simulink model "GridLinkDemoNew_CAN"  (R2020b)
settings: Solver=FixedStepDiscrete  StartTime=0.0  StopTime=inf  RelTol=1e-3  EnableMultiTasking=on
InitFcn:
  | clc
  | close all
  | f_mod = 50000;
  | f_mod1 = 50*1e3; %[12 24 36 48 72 84 96 144]*1e3; %[18 36 48 72 84 96 144]*1e3;%
  | 
  | 
  | %%
  | 
  | 
  |             Tmod1 = 1/f_mod1;
  |             Tmod = 1/f_mod;
  |             Tc = Tmod1;
  |             Tsw=Tc;
  | 
  | warning off
  | f_sig = 60;
  | 
  | U_ac = 10;
  | U_dc = 20;
  | Ts= 0.01*Tsw;
  | 
  | Fc=50000
  | Fc1=1000
  | 
  | 
  | CounterCut_Outer=2000
  | 
  | 
  | INNER_PWM=1000
  | OUTER_PWM=50000
undefined symbols (not defined in the file): A, ADCIN0, ADCIN1, ADCINA0, ADCINB0, bit, Compare, conversion, DCAEVT1, DCAEVT1FILT, Digital, Down, ended, Event, Filtered, GPTRIP1SEL, GPTRIP2SEL, hex2dec, identifier, input, Module, Newinv, of, Single, SPS_EMT_TAPAS_2018b, Standard, start, Trip, TZ1, TZ2, Up, version, Zone
libraries: tiiqmathlib x63, c2802xlib x25, c2837xDlib x5, c280xlib x5, c28xdmclib x2, svdutilitieslib x1, c2000lib x1, canmsglib x1, simulink x1
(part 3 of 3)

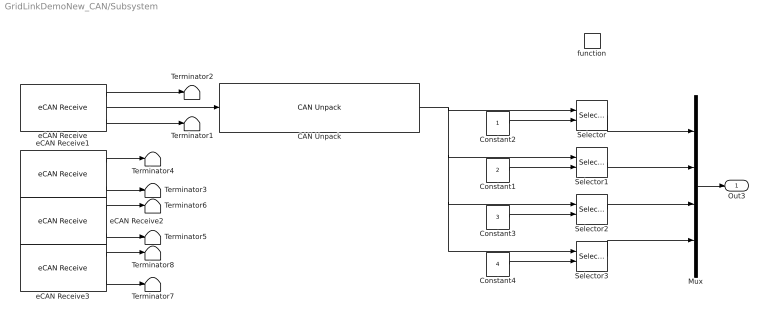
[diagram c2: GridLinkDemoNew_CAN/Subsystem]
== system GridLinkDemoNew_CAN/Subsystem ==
  function : TriggerPort  TriggerType=function-call  VariantControl=Variant
  CAN Unpack : canmsglib/CAN Unpack  MsgList=(none)  MsgName=CAN Msg  MsgIDType=Standard (11-bit identifier)  MsgIdentifier=hex2dec('01A')  MsgLength=4  SignalInfo={}  IDPort=off  TimestampPort=off  ErrorPort=off  RemotePort=off  LengthPort=off  StatusPort=off  ApplyMinMax=off
  Constant1 : Constant  Value=2  OutDataTypeStr=Inherit: Inherit via back propagation
  Constant2 : Constant  OutDataTypeStr=Inherit: Inherit via back propagation
  Constant3 : Constant  Value=3  OutDataTypeStr=Inherit: Inherit via back propagation
  Constant4 : Constant  Value=4  OutDataTypeStr=Inherit: Inherit via back propagation
  Mux : Mux
  Selector{,1..3} (4 alike) : Selector  InputPortWidth=4  IndexOptions=Index vector (port)  Indices=1  OutputSizes=1
  Terminator{1..8} (8 alike) : Terminator
  eCAN Receive : c280xlib/eCAN Receive  chipFamily=C280x  useModule=eCAN_B  mailboxNo=2  messageID=hex2dec('01A')  messageType=Standard (11-bit identifier)  sampleTime=-1  dataType=CAN_MESSAGE_TYPE  initValue=0  outputMessageLength=on  outputMessageTimeStamp=off  postInterrupt=on  interruptLine=0
  eCAN Receive1 : c280xlib/eCAN Receive  Commented=on  chipFamily=C280x  useModule=eCAN_B  mailboxNo=3  messageID=hex2dec('02A')  messageType=Standard (11-bit identifier)  sampleTime=-1  dataType=uint16  initValue=0  outputMessageLength=on  outputMessageTimeStamp=off  postInterrupt=on  interruptLine=0
  eCAN Receive2 : c280xlib/eCAN Receive  Commented=on  chipFamily=C280x  useModule=eCAN_B  mailboxNo=4  messageID=hex2dec('03A')  messageType=Standard (11-bit identifier)  sampleTime=-1  dataType=uint16  initValue=0  outputMessageLength=on  outputMessageTimeStamp=off  postInterrupt=on  interruptLine=0
  eCAN Receive3 : c280xlib/eCAN Receive  Commented=on  chipFamily=C280x  useModule=eCAN_B  mailboxNo=5  messageID=hex2dec('04A')  messageType=Standard (11-bit identifier)  sampleTime=-1  dataType=uint16  initValue=0  outputMessageLength=on  outputMessageTimeStamp=off  postInterrupt=on  interruptLine=0
  Out3 : Outport  VectorParamsAs1DForOutWhenUnconnected=off
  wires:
  eCAN Receive/1 -> Terminator2/1
  Constant2/1 -> Selector/2
  eCAN Receive/3 -> Terminator1/1
  eCAN Receive1/3 -> Terminator3/1
  Constant1/1 -> Selector1/2
  Selector1/1 -> Mux/2
  eCAN Receive1/1 -> Terminator4/1
  Constant3/1 -> Selector2/2
  eCAN Receive2/3 -> Terminator5/1
  Selector2/1 -> Mux/3
  eCAN Receive2/1 -> Terminator6/1
  Constant4/1 -> Selector3/2
  eCAN Receive3/3 -> Terminator7/1
  Selector3/1 -> Mux/4
  eCAN Receive3/1 -> Terminator8/1
  Mux/1 -> Out3/1
  Selector/1 -> Mux/1
  CAN Unpack/1 -> Selector3/1, Selector2/1, Selector1/1, Selector/1
  eCAN Receive/2 -> CAN Unpack/1

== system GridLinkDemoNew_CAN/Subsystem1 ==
  ePWM : c2802xlib/ePWM  PwmType=C2000_Type4  useModule=ePWM8  ePWMxLINKTBPRD=Not Linked  periodUnits=Clock cycles  timerSource=Specify via dialog  timerPeriod_clk=250  timerPeriod_sec=0.0001  tbshadow=Counter equals to zero  countingMode=Up-Down  phaseActiveEnable=Disable  phaseDirection=Count down after sync  phaseActive=0  synchronizationEnable=off  dcaevt1Sync=off  dcbevt1Sync=off  synchronizationOption=Disable  perSynchronizationOption=Counter equals to period (CTR=PRD)  clockPrescale=1  HSclockPrescale=1  enswap=off  ePWMxAStatus=on  ePWMxAactionLogic1=Do nothing  ePWMxAactionLogic2=Do nothing  ePWMxAactionLogic3=Set  ePWMxAactionLogic4=Clear  ePWMxAactionLogic5=Do nothing  ePWMxAactionLogic6=Do nothing  ePWMxACSFenable=off  ePWMxACSFvalue=Forcing disable  ePWMxASFreload=Zero  ePWMxBStatus=on  ePWMxBactionLogic1=Do nothing  ePWMxBactionLogic2=Do nothing  ePWMxBactionLogic3=Do nothing  ePWMxBactionLogic4=Do nothing  ePWMxBactionLogic5=Do nothing  ePWMxBactionLogic6=Do nothing  ePWMxBCSFenable=off  ePWMxBCSFvalue=Forcing disable  ePWMxBSFreload=Zero  ePWNxBOutWay=off  ePWMxLINKCMPA=Not Linked  CMPAUnits=Clock cycles  CMPASource=Specify via dialog  CMPAValue_per=50  CMPAValue_clk=10  enCMPAshadow=Counter equals to zero (CTR=Zero)  ePWMxLINKCMPB=Not Linked  CMPBUnits=Clock cycles  CMPBSource=Specify via dialog  CMPBValue_per=50  CMPBValue_clk=0  enCMPBshadow=Counter equals to zero (CTR=Zero)  ePWMxLINKCMPC=Not Linked  CMPCUnits=Clock cycles  CMPCSource=Specify via dialog  CMPCValue_per=50  CMPCValue_clk=0  enCMPCshadow=Counter equals to zero (CTR=Zero)  ePWMxLINKCMPD=Not Linked  CMPDUnits=Clock cycles  CMPDSource=Specify via dialog  CMPDValue_per=50  CMPDValue_clk=0  enCMPDshadow=Counter equals to zero (CTR=Zero)  enableDBePWMxA=off  enableDBePWMxB=off  enhalfcycle=off  DBpolarity=Active high (AH)  DBedgeDelay=Positive  DBSource_ePWMxA=ePWMxA  DBSource_ePWMxB=ePWMxA  DBPeriodUnits=Clock cycles  DBperiodSource=Specify via dialog  REDperiod=0  FEDperiod=0  REDperiod_sec=0  FEDperiod_sec=0  LoadModeDBRED=Immediate without using shadow  LoadModeDBFED=Immediate without using shadow  adcstartModuleA=off  adcrequestEventA=First event  adcstartEventA=Digital Compare Module A Event 1 start of conversion (DCAEVT1.soc)  adcstartEventA_type2=Counter equals to period (CTR=PRD)  adcstartModuleB=off  adcrequestEventB=First event  adcstartEventB=Counter equals to zero (CTR=Zero)  adcstartEventB_type2=Counter equals to zero (CTR=Zero)  intEn=on  intPrd=Third event  intSel=Counter equals to zero (CTR=Zero)  intSel_type2=Counter equals to zero (CTR=Zero)  hrpe=off  enHRPWM=off  HRPWM_LoadMode=Counter equals to period (CTR=PRD)  HRPWM_CTLMode=Duty or Period control mode  HRPWM_EDGMode=Both edge  hrpeb=off  enHRPWMB=off  HRPWM_LoadModeB=Counter equals to zero (CTR=ZERO)  HRPWM_CTLModeB=Duty or Period control mode  HRPWM_EDGModeB=Both edge  enHRDBRED=off  enHRDBFED=off  enSFO=on  enautoconv=on  chopperEnable=off  chopperFrequency=1  chopperFirstwidth=1  chopperDuty=12.5%  tripZonesource=Specify via dialog  tzselOSHT1=off  tzselOSHT2=off  tzselOSHT3=off  tzselOSHDCAEV1=off  tzselOSHDCBEV1=off  tzselCBC1=off  tzselCBC2=off  tzselCBC3=off  tzselCBCDCAEV2=off  tzselCBCDCBEV2=off  tzselOSHT4=off  tzselOSHT5=off  tzselOSHT6=off  tzselCBC4=off  tzselCBC5=off  tzselCBC6=off  enTzOstIntr=off  enTzCbcIntr=off  enTzDCAEVT1Intr=off  enTzDCAEVT2Intr=off  enTzDCBEVT1Intr=off  enTzDCBEVT2Intr=off  ePWMxAforced=No action  ePWMxBforced=No action  DCAEVT1forced=No action  DCBEVT1forced=No action  DCAEVT2forced=No action  DCBEVT2forced=No action  dcah=Trip Zone 1 input (TZ1)  dcal=Trip Zone 2 input (TZ2)  dcbh=Trip Zone 1 input (TZ1)  dcbl=Trip Zone 2 input (TZ2)  dcah_type2=GPTRIP1SEL/(TZ1)  dcal_type2=GPTRIP2SEL/(TZ2)  dcbh_type2=GPTRIP1SEL/(TZ1)  dcbl_type2=GPTRIP2SEL/(TZ2)  gendcaevt1=Event disabled  gendcaevt2=Event disabled  gendcbevt1=Event disabled  gendcbevt2=Event disabled  dcaevt1src=DCAEVT1 with sync  dcaevt2src=DCAEVT2 with sync  dcbevt1src=DCBEVT1 with sync  dcbevt2src=DCBEVT2 with sync  pulsesel=Counter equals to zero (CTR=Zero)  blankinv=off  blankoffset=0  blankwidth=0  evsrcsel=Filtered version of DCAEVT1 (DCAEVT1FILT)  encape=off

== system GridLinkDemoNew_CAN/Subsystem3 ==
  note: counter +=
  note: Reset counter
  function : TriggerPort  TriggerType=function-call  VariantControl=Variant
  Data Store Read1 : DataStoreRead  DataStoreName=CounterCut
  Data Store Read2 : DataStoreRead  DataStoreName=Counter
  If : If  NumInputs=2  IfExpression=u1 >= u2
  If Action Subsystem : Subsystem  TreatAsAtomicUnit=on
  If Action Subsystem1 : Subsystem  TreatAsAtomicUnit=on
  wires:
  Data Store Read2/1 -> If/1
  Data Store Read1/1 -> If/2
  If/2 -> If Action Subsystem1/Action
  If/1 -> If Action Subsystem/Action

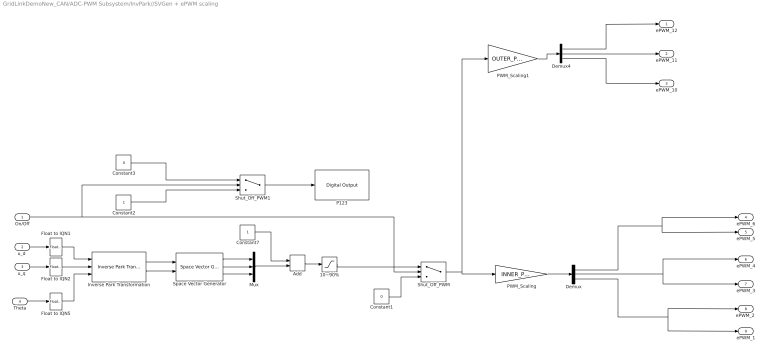
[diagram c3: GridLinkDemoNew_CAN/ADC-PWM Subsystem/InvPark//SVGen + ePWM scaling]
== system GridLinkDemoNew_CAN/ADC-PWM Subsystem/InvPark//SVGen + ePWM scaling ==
  On/Off : Inport
  "u_d " : Inport  Port=2
  "u_q " : Inport  Port=3
  Theta : Inport  Port=4
  10~90% : Saturate  UpperLimit=1.8  LowerLimit=0.2  OutDataTypeStr=Inherit: Inherit via back propagation
  Add : Sum
  Constant1 : Constant  Value=0  OutDataTypeStr=Inherit: Inherit via back propagation
  Constant2 : Constant  OutDataTypeStr=boolean
  Constant3 : Constant  Value=0  OutDataTypeStr=boolean
  Constant7 : Constant  OutDataTypeStr=Inherit: Inherit via back propagation
  Demux : Demux  Outputs=3
  Demux4 : Demux  Outputs=3
  Float to IQN1 : tiiqmathlib/Float to IQN  Q_value=16
  Float to IQN2 : tiiqmathlib/Float to IQN  Q_value=16
  Float to IQN5 : tiiqmathlib/Float to IQN  Q_value=16
  Inverse Park Transformation : c28xdmclib/Inverse Park Transformation
  Mux : Mux  Inputs=3
  P123 : c2837xDlib/Digital Output  GPIO_Number=GPIO112~GPIO119  GPIO_Bit0=off  GPIO_BIT0_Toggle=on  GPIO_Bit1=off  GPIO_BIT1_Toggle=on  GPIO_Bit2=off  GPIO_BIT2_Toggle=off  GPIO_Bit3=off  GPIO_BIT3_Toggle=off  GPIO_Bit4=off  GPIO_BIT4_Toggle=off  GPIO_Bit5=off  GPIO_BIT5_Toggle=on  GPIO_Bit6=off  GPIO_BIT6_Toggle=off  GPIO_Bit7=on  GPIO_BIT7_Toggle=off
  PWM_Scaling : Gain  Gain=INNER_PWM/2  ParamDataTypeStr=Inherit: Inherit from 'Gain'  OutDataTypeStr=Inherit: Inherit via back propagation
  PWM_Scaling1 : Gain  Gain=OUTER_PWM/2  ParamDataTypeStr=Inherit: Inherit from 'Gain'  OutDataTypeStr=Inherit: Inherit via back propagation
  Shut_Off_PWM : Switch  Criteria=u2 > Threshold  OutDataTypeStr=Inherit: Inherit via back propagation
  Shut_Off_PWM1 : Switch  Criteria=u2 > Threshold  OutDataTypeStr=Inherit: Inherit via back propagation
  Space Vector Generator : c28xdmclib/Space Vector Generator
  ePWM_12 : Outport  VectorParamsAs1DForOutWhenUnconnected=off
  ePWM_11 : Outport  Port=2  VectorParamsAs1DForOutWhenUnconnected=off
  ePWM_10 : Outport  Port=3  VectorParamsAs1DForOutWhenUnconnected=off
  ePWM_6 : Outport  Port=4  VectorParamsAs1DForOutWhenUnconnected=off
  ePWM_5 : Outport  Port=5  VectorParamsAs1DForOutWhenUnconnected=off
  ePWM_4 : Outport  Port=6  VectorParamsAs1DForOutWhenUnconnected=off
  ePWM_3 : Outport  Port=7  VectorParamsAs1DForOutWhenUnconnected=off
  "ePWM_2 " : Outport  Port=8  VectorParamsAs1DForOutWhenUnconnected=off
  ePWM_1 : Outport  Port=9  VectorParamsAs1DForOutWhenUnconnected=off
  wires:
  Float to IQN5/1 -> Inverse Park Transformation/3
  Theta/1 -> Float to IQN5/1
  "u_d "/1 -> Float to IQN1/1
  Space Vector Generator/3 -> Mux/3
  Space Vector Generator/2 -> Mux/2
  Space Vector Generator/1 -> Mux/1
  10~90%/1 -> Shut_Off_PWM/1
  Inverse Park Transformation/1 -> Space Vector Generator/1
  Mux/1 -> Add/2
  Add/1 -> 10~90%/1
  Inverse Park Transformation/2 -> Space Vector Generator/2
  Constant7/1 -> Add/1
  "u_q "/1 -> Float to IQN2/1
  Constant1/1 -> Shut_Off_PWM/3
  On/Off/1 -> Shut_Off_PWM1/2, Shut_Off_PWM/2
  Shut_Off_PWM1/1 -> P123/1
  Constant2/1 -> Shut_Off_PWM1/3
  Constant3/1 -> Shut_Off_PWM1/1
  Float to IQN1/1 -> Inverse Park Transformation/1
  Float to IQN2/1 -> Inverse Park Transformation/2
  Demux4/1 -> ePWM_12/1
  Demux4/3 -> ePWM_10/1
  Demux4/2 -> ePWM_11/1
  Shut_Off_PWM/1 -> PWM_Scaling/1, PWM_Scaling1/1
  PWM_Scaling1/1 -> Demux4/1
  PWM_Scaling/1 -> Demux/1
  Demux/1 -> ePWM_5/1, ePWM_6/1
  Demux/2 -> ePWM_4/1, ePWM_3/1
  Demux/3 -> "ePWM_2 "/1, ePWM_1/1

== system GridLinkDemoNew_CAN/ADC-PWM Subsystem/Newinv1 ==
  note: Input: uint16 Output: sfix32_En16
  note: voltage amplified by 100: e.g., 12 V => 1200
  A4 : Inport  OutDataTypeStr=uint16  PortDimensions=1
  A5 : Inport  Port=2  OutDataTypeStr=uint16  PortDimensions=1
  A6 : Inport  Port=3  OutDataTypeStr=uint16  PortDimensions=1
  B0 : Inport  Port=4  OutDataTypeStr=uint16  PortDimensions=1
  B1 : Inport  Port=5  OutDataTypeStr=uint16  PortDimensions=1
  B2 : Inport  Port=6  OutDataTypeStr=uint16  PortDimensions=1
  theta : Inport  Port=7
  Current scaling + Clarke/Park : Subsystem
  Voltage scaling + Clarke/Park : Subsystem
  Vd : Outport  PortDimensions=1  VectorParamsAs1DForOutWhenUnconnected=off
  Vq : Outport  Port=2  PortDimensions=1  VectorParamsAs1DForOutWhenUnconnected=off
  Id : Outport  Port=3  PortDimensions=1  VectorParamsAs1DForOutWhenUnconnected=off
  Iq : Outport  Port=4  PortDimensions=1  VectorParamsAs1DForOutWhenUnconnected=off
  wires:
  A5/1 -> Voltage scaling + Clarke/Park/2(V_ADC_2)
  Voltage scaling + Clarke/Park/2(V_q (ADC)) -> Vq/1
  B0/1 -> Current scaling + Clarke/Park/1(I_ADC_1)
  A4/1 -> Voltage scaling + Clarke/Park/1(V_ADC_1)
  A6/1 -> Voltage scaling + Clarke/Park/3(V_ADC_3)
  B2/1 -> Current scaling + Clarke/Park/3(I_ADC_3)
  B1/1 -> Current scaling + Clarke/Park/2(I_ADC_2)
  [theta] -> Voltage scaling + Clarke/Park/4(Theta)
  [theta] -> Current scaling + Clarke/Park/4(Theta)
  theta/1 -> [theta]
  Current scaling + Clarke/Park/1(I_d (ADC)) -> Id/1
  Current scaling + Clarke/Park/2(I_q (ADC)) -> Iq/1
  Voltage scaling + Clarke/Park/1(V_d (ADC)) -> Vd/1

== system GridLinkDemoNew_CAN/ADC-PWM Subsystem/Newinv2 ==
  note: Input: uint16 Output: sfix32_En16
  note: voltage amplified by 100: e.g., 12 V => 1200
  A4 : Inport  OutDataTypeStr=uint16  PortDimensions=1
  A5 : Inport  Port=2  OutDataTypeStr=uint16  PortDimensions=1
  A6 : Inport  Port=3  OutDataTypeStr=uint16  PortDimensions=1
  B0 : Inport  Port=4  OutDataTypeStr=uint16  PortDimensions=1
  B1 : Inport  Port=5  OutDataTypeStr=uint16  PortDimensions=1
  B2 : Inport  Port=6  OutDataTypeStr=uint16  PortDimensions=1
  theta : Inport  Port=7
  Current scaling + Clarke/Park : Subsystem
  Voltage scaling + Clarke/Park : Subsystem
  Vd : Outport  PortDimensions=1  VectorParamsAs1DForOutWhenUnconnected=off
  Vq : Outport  Port=2  PortDimensions=1  VectorParamsAs1DForOutWhenUnconnected=off
  Id : Outport  Port=3  PortDimensions=1  VectorParamsAs1DForOutWhenUnconnected=off
  Iq : Outport  Port=4  PortDimensions=1  VectorParamsAs1DForOutWhenUnconnected=off
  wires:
  A5/1 -> Voltage scaling + Clarke/Park/2(V_ADC_2)
  Voltage scaling + Clarke/Park/2(V_q (ADC)) -> Vq/1
  B0/1 -> Current scaling + Clarke/Park/1(I_ADC_1)
  A4/1 -> Voltage scaling + Clarke/Park/1(V_ADC_1)
  A6/1 -> Voltage scaling + Clarke/Park/3(V_ADC_3)
  B2/1 -> Current scaling + Clarke/Park/3(I_ADC_3)
  B1/1 -> Current scaling + Clarke/Park/2(I_ADC_2)
  [theta] -> Voltage scaling + Clarke/Park/4(Theta)
  [theta] -> Current scaling + Clarke/Park/4(Theta)
  theta/1 -> [theta]
  Current scaling + Clarke/Park/1(I_d (ADC)) -> Id/1
  Current scaling + Clarke/Park/2(I_q (ADC)) -> Iq/1
  Voltage scaling + Clarke/Park/1(V_d (ADC)) -> Vd/1

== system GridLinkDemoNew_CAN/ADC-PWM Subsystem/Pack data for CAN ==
  In1 : Inport
  In2 : Inport  Port=2
  In3 : Inport  Port=3
  In4 : Inport  Port=4
  Byte Pack2 : svdutilitieslib/Byte Pack  maskPackedDataType=uint16  datatypes={'uint16' 'uint16' 'uint16' 'uint16'}  byteAlign=2  blockPlatform=tic2000
  Data Type Conversion7 : DataTypeConversion  OutDataTypeStr=uint16
  Demux4 : Demux
  Mux6 : Mux
  Output : Outport  OutDataTypeStr=uint16  VectorParamsAs1DForOutWhenUnconnected=off
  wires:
  Mux6/1 -> Data Type Conversion7/1
  In1/1 -> Mux6/1
  Data Type Conversion7/1 -> Demux4/1
  In2/1 -> Mux6/2
  In4/1 -> Mux6/4
  In3/1 -> Mux6/3
  Byte Pack2/1 -> Output/1
  Demux4/1 -> Byte Pack2/1
  Demux4/2 -> Byte Pack2/2
  Demux4/3 -> Byte Pack2/3
  Demux4/4 -> Byte Pack2/4

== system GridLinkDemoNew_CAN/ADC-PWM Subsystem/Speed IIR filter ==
  Speed : Inport
  Add : Sum  Inputs=+-
  Add1 : Sum
  Constant1 : Constant  OutDataTypeStr=fixdt(1,32,16)
  Constant2 : Constant  Value=.01  OutDataTypeStr=fixdt(1,32,16)
  Product : Product
  Product1 : Product
  Unit Delay : UnitDelay  SampleTime=-1  HasFrameUpgradeWarning=on
  Filtered speed : Outport  VectorParamsAs1DForOutWhenUnconnected=off
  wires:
  Product1/1 -> Add1/2
  Unit Delay/1 -> Product1/2
  Add/1 -> Product1/1
  Product/1 -> Add1/1
  Constant2/1 -> Add/2, Product/2
  Constant1/1 -> Add/1
  Add1/1 -> Filtered speed/1, Unit Delay/1
  Speed/1 -> Product/1

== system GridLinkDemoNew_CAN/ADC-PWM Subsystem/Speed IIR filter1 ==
  Speed : Inport
  Add : Sum  Inputs=+-
  Add1 : Sum
  Constant1 : Constant  OutDataTypeStr=fixdt(1,32,16)
  Constant2 : Constant  Value=.01  OutDataTypeStr=fixdt(1,32,16)
  Product : Product
  Product1 : Product
  Unit Delay : UnitDelay  SampleTime=-1  HasFrameUpgradeWarning=on
  Filtered speed : Outport  VectorParamsAs1DForOutWhenUnconnected=off
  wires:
  Product1/1 -> Add1/2
  Unit Delay/1 -> Product1/2
  Add/1 -> Product1/1
  Product/1 -> Add1/1
  Constant2/1 -> Add/2, Product/2
  Constant1/1 -> Add/1
  Add1/1 -> Filtered speed/1, Unit Delay/1
  Speed/1 -> Product/1

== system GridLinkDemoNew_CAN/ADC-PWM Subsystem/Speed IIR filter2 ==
  Speed : Inport
  Add : Sum  Inputs=+-
  Add1 : Sum
  Constant1 : Constant  OutDataTypeStr=fixdt(1,32,16)
  Constant2 : Constant  Value=.01  OutDataTypeStr=fixdt(1,32,16)
  Product : Product
  Product1 : Product
  Unit Delay : UnitDelay  SampleTime=-1  HasFrameUpgradeWarning=on
  Filtered speed : Outport  VectorParamsAs1DForOutWhenUnconnected=off
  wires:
  Product1/1 -> Add1/2
  Unit Delay/1 -> Product1/2
  Add/1 -> Product1/1
  Product/1 -> Add1/1
  Constant2/1 -> Add/2, Product/2
  Constant1/1 -> Add/1
  Add1/1 -> Filtered speed/1, Unit Delay/1
  Speed/1 -> Product/1

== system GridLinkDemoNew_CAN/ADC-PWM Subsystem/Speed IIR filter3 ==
  Speed : Inport
  Add : Sum  Inputs=+-
  Add1 : Sum
  Constant1 : Constant  OutDataTypeStr=fixdt(1,32,16)
  Constant2 : Constant  Value=.01  OutDataTypeStr=fixdt(1,32,16)
  Product : Product
  Product1 : Product
  Unit Delay : UnitDelay  SampleTime=-1  HasFrameUpgradeWarning=on
  Filtered speed : Outport  VectorParamsAs1DForOutWhenUnconnected=off
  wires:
  Product1/1 -> Add1/2
  Unit Delay/1 -> Product1/2
  Add/1 -> Product1/1
  Product/1 -> Add1/1
  Constant2/1 -> Add/2, Product/2
  Constant1/1 -> Add/1
  Add1/1 -> Filtered speed/1, Unit Delay/1
  Speed/1 -> Product/1

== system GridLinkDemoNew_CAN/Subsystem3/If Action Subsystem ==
  Action Port : ActionPort  ActionPortLabel=if(u1 >= u2)
  Constant : Constant  Value=0  OutDataTypeStr=single
  Data Store Write1 : DataStoreWrite  DataStoreName=Counter
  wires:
  Constant/1 -> Data Store Write1/1

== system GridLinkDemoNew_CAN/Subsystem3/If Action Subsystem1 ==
  Action Port : ActionPort  ActionPortLabel=else
  Data Store Read1 : DataStoreRead  DataStoreName=Counter
  Data Store Write1 : DataStoreWrite  DataStoreName=Counter
  Increment Stored Integer1 : simulink/Additional Math & Discrete/Additional Math: Increment - Decrement/Increment Stored Integer
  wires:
  Data Store Read1/1 -> Increment Stored Integer1/1
  Increment Stored Integer1/1 -> Data Store Write1/1

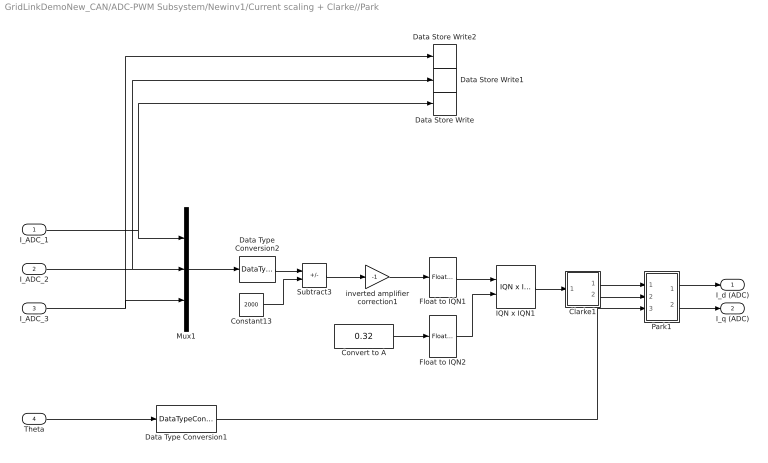
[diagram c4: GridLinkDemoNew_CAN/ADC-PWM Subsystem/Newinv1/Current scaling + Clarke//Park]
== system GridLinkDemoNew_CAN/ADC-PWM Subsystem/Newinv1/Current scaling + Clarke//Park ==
  I_ADC_1 : Inport
  I_ADC_2 : Inport  Port=2
  I_ADC_3 : Inport  Port=3
  Theta : Inport  Port=4
  Clarke1 : Subsystem
  Constant13 : Constant  Value=2000  OutDataTypeStr=single
  Convert to A : Constant  Value=0.32  OutDataTypeStr=single
  Data Store Write : DataStoreWrite  DataStoreName=I_s_A
  Data Store Write1 : DataStoreWrite  DataStoreName=I_s_B
  Data Store Write2 : DataStoreWrite  DataStoreName=I_s_C
  Data Type Conversion1 : DataTypeConversion
  Data Type Conversion2 : DataTypeConversion  OutDataTypeStr=single
  Float to IQN1 : tiiqmathlib/Float to IQN  Q_value=16
  Float to IQN2 : tiiqmathlib/Float to IQN  Q_value=16
  IQN x IQN1 : tiiqmathlib/IQN x IQN  multiplyOption=Multiply
  Mux1 : Mux  Inputs=3
  Park1 : Subsystem
  Subtract3 : Sum  Inputs=+-
  inverted amplifier correction1 : Gain  Gain=-1  ParamDataTypeStr=Inherit: Inherit from 'Gain'
  I_d (ADC) : Outport  VectorParamsAs1DForOutWhenUnconnected=off
  I_q (ADC) : Outport  Port=2  VectorParamsAs1DForOutWhenUnconnected=off
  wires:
  Convert to A/1 -> Float to IQN2/1
  Theta/1 -> Data Type Conversion1/1
  Park1/2(q) -> I_q (ADC)/1
  Clarke1/1(Alpha) -> Park1/1(Alpha)
  Mux1/1 -> Data Type Conversion2/1
  inverted amplifier correction1/1 -> Float to IQN1/1
  Data Type Conversion2/1 -> Subtract3/1
  Constant13/1 -> Subtract3/2
  Subtract3/1 -> inverted amplifier correction1/1
  IQN x IQN1/1 -> Clarke1/1(ABC)
  Float to IQN1/1 -> IQN x IQN1/1
  Park1/1(d) -> I_d (ADC)/1
  Float to IQN2/1 -> IQN x IQN1/2
  Data Type Conversion1/1 -> Park1/3(theta)
  Clarke1/2(Beta) -> Park1/2(Beta)
  I_ADC_2/1 -> Data Store Write1/1, Mux1/2
  I_ADC_3/1 -> Data Store Write2/1, Mux1/3
  I_ADC_1/1 -> Data Store Write/1, Mux1/1

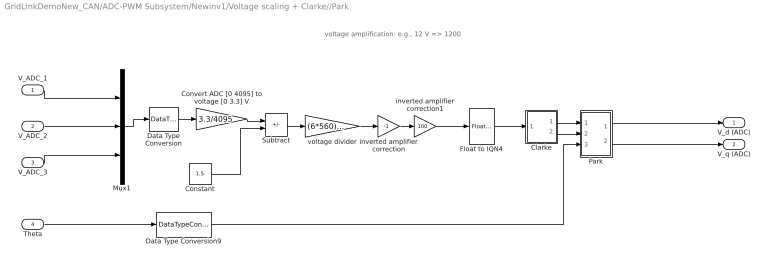
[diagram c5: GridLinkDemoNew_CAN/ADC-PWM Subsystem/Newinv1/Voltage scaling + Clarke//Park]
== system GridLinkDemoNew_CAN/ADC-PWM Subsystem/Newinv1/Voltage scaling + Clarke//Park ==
  note: voltage amplification: e.g., 12 V => 1200
  V_ADC_1 : Inport
  V_ADC_2 : Inport  Port=2
  V_ADC_3 : Inport  Port=3
  Theta : Inport  Port=4
  Clarke : Subsystem
  Constant : Constant  Value=1.5
  Convert ADC [0 4095] to voltage [0 3.3] V : Gain  Gain=3.3/4095  ParamDataTypeStr=Inherit: Inherit from 'Gain'  OutDataTypeStr=single
  Data Type Conversion : DataTypeConversion  OutDataTypeStr=single
  Data Type Conversion9 : DataTypeConversion
  Float to IQN4 : tiiqmathlib/Float to IQN  Q_value=16
  Mux1 : Mux  Inputs=3
  Park : Subsystem
  Subtract : Sum  Inputs=+-
  inverted amplifier correction : Gain  Gain=-1  ParamDataTypeStr=Inherit: Inherit from 'Gain'
  inverted amplifier correction1 : Gain  Gain=100  ParamDataTypeStr=Inherit: Inherit from 'Gain'
  voltage divider : Gain  Gain=(6*560)/(4.7+5.6)  ParamDataTypeStr=Inherit: Inherit from 'Gain'  OutDataTypeStr=single
  V_d (ADC) : Outport  VectorParamsAs1DForOutWhenUnconnected=off
  V_q (ADC) : Outport  Port=2  VectorParamsAs1DForOutWhenUnconnected=off
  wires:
  Data Type Conversion9/1 -> Park/3(theta)
  Clarke/1(Alpha) -> Park/1(Alpha)
  Mux1/1 -> Data Type Conversion/1
  V_ADC_2/1 -> Mux1/2
  V_ADC_1/1 -> Mux1/1
  Clarke/2(Beta) -> Park/2(Beta)
  voltage divider/1 -> inverted amplifier correction/1
  Park/1(d) -> V_d (ADC)/1
  Park/2(q) -> V_q (ADC)/1
  V_ADC_3/1 -> Mux1/3
  Theta/1 -> Data Type Conversion9/1
  Float to IQN4/1 -> Clarke/1(ABC)
  Data Type Conversion/1 -> Convert ADC [0 4095] to voltage [0 3.3] V/1
  inverted amplifier correction1/1 -> Float to IQN4/1
  inverted amplifier correction/1 -> inverted amplifier correction1/1
  Subtract/1 -> voltage divider/1
  Convert ADC [0 4095] to voltage [0 3.3] V/1 -> Subtract/1
  Constant/1 -> Subtract/2

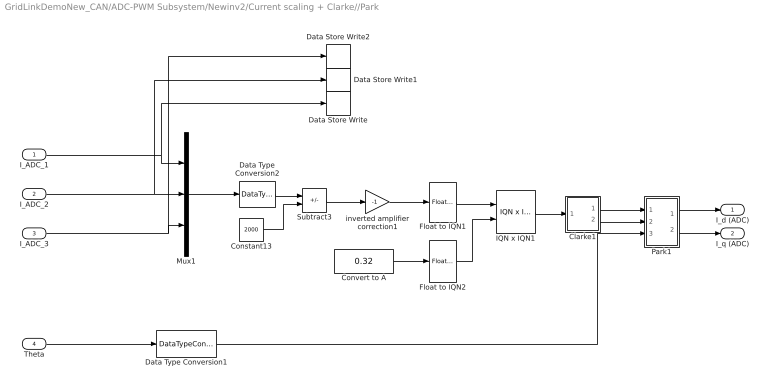
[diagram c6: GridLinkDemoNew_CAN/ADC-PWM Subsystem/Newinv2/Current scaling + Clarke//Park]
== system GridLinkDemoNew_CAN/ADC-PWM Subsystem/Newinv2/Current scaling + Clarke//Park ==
  I_ADC_1 : Inport
  I_ADC_2 : Inport  Port=2
  I_ADC_3 : Inport  Port=3
  Theta : Inport  Port=4
  Clarke1 : Subsystem
  Constant13 : Constant  Value=2000  OutDataTypeStr=single
  Convert to A : Constant  Value=0.32  OutDataTypeStr=single
  Data Store Write : DataStoreWrite  DataStoreName=I_o_A
  Data Store Write1 : DataStoreWrite  DataStoreName=I_o_B
  Data Store Write2 : DataStoreWrite  DataStoreName=I_o_C
  Data Type Conversion1 : DataTypeConversion
  Data Type Conversion2 : DataTypeConversion  OutDataTypeStr=single
  Float to IQN1 : tiiqmathlib/Float to IQN  Q_value=16
  Float to IQN2 : tiiqmathlib/Float to IQN  Q_value=16
  IQN x IQN1 : tiiqmathlib/IQN x IQN  multiplyOption=Multiply
  Mux1 : Mux  Inputs=3
  Park1 : Subsystem
  Subtract3 : Sum  Inputs=+-
  inverted amplifier correction1 : Gain  Gain=-1  ParamDataTypeStr=Inherit: Inherit from 'Gain'
  I_d (ADC) : Outport  VectorParamsAs1DForOutWhenUnconnected=off
  I_q (ADC) : Outport  Port=2  VectorParamsAs1DForOutWhenUnconnected=off
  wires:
  Convert to A/1 -> Float to IQN2/1
  Theta/1 -> Data Type Conversion1/1
  Park1/2(q) -> I_q (ADC)/1
  I_ADC_3/1 -> Data Store Write2/1, Mux1/3
  I_ADC_2/1 -> Data Store Write1/1, Mux1/2
  Clarke1/1(Alpha) -> Park1/1(Alpha)
  I_ADC_1/1 -> Data Store Write/1, Mux1/1
  inverted amplifier correction1/1 -> Float to IQN1/1
  Data Type Conversion2/1 -> Subtract3/1
  Constant13/1 -> Subtract3/2
  Subtract3/1 -> inverted amplifier correction1/1
  Float to IQN1/1 -> IQN x IQN1/1
  Park1/1(d) -> I_d (ADC)/1
  Float to IQN2/1 -> IQN x IQN1/2
  Data Type Conversion1/1 -> Park1/3(theta)
  Clarke1/2(Beta) -> Park1/2(Beta)
  Mux1/1 -> Data Type Conversion2/1
  IQN x IQN1/1 -> Clarke1/1(ABC)

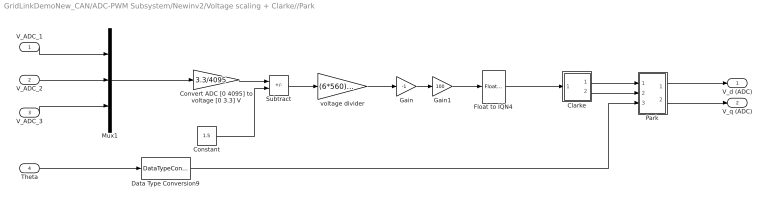
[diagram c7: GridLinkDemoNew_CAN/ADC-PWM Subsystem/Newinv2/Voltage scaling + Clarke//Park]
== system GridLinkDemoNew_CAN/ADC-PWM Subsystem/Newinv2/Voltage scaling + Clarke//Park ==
  V_ADC_1 : Inport
  V_ADC_2 : Inport  Port=2
  V_ADC_3 : Inport  Port=3
  Theta : Inport  Port=4
  Clarke : Subsystem
  Constant : Constant  Value=1.5
  Convert ADC [0 4095] to voltage [0 3.3] V : Gain  Gain=3.3/4095  ParamDataTypeStr=Inherit: Inherit from 'Gain'  OutDataTypeStr=single
  Data Type Conversion9 : DataTypeConversion
  Float to IQN4 : tiiqmathlib/Float to IQN  Q_value=16
  Gain : Gain  Gain=-1
  Gain1 : Gain  Gain=100
  Mux1 : Mux  Inputs=3
  Park : Subsystem
  Subtract : Sum  Inputs=+-
  voltage divider : Gain  Gain=(6*560)/(4.7+5.6)  ParamDataTypeStr=Inherit: Inherit from 'Gain'  OutDataTypeStr=single
  V_d (ADC) : Outport  VectorParamsAs1DForOutWhenUnconnected=off
  V_q (ADC) : Outport  Port=2  VectorParamsAs1DForOutWhenUnconnected=off
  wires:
  Data Type Conversion9/1 -> Park/3(theta)
  Clarke/1(Alpha) -> Park/1(Alpha)
  V_ADC_2/1 -> Mux1/2
  Float to IQN4/1 -> Clarke/1(ABC)
  V_ADC_1/1 -> Mux1/1
  Clarke/2(Beta) -> Park/2(Beta)
  Park/1(d) -> V_d (ADC)/1
  Park/2(q) -> V_q (ADC)/1
  V_ADC_3/1 -> Mux1/3
  Theta/1 -> Data Type Conversion9/1
  voltage divider/1 -> Gain/1
  Mux1/1 -> Convert ADC [0 4095] to voltage [0 3.3] V/1
  Gain1/1 -> Float to IQN4/1
  Gain/1 -> Gain1/1
  Convert ADC [0 4095] to voltage [0 3.3] V/1 -> Subtract/1
  Subtract/1 -> voltage divider/1
  Constant/1 -> Subtract/2

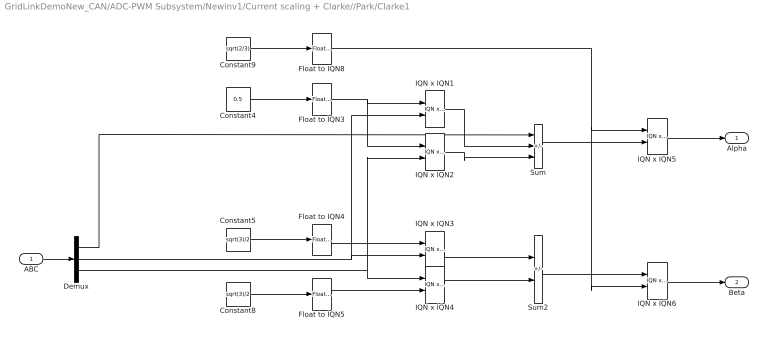
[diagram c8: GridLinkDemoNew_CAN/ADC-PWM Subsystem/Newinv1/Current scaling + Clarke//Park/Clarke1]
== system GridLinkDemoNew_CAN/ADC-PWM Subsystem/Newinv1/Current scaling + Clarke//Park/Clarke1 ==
  ABC : Inport
  Constant4 : Constant  Value=0.5  OutDataTypeStr=single
  Constant5 : Constant  Value=sqrt(3)/2  OutDataTypeStr=single
  Constant8 : Constant  Value=sqrt(3)/2  OutDataTypeStr=single
  Constant9 : Constant  Value=sqrt(2/3)  OutDataTypeStr=single
  Demux : Demux  Outputs=3
  Float to IQN{3..5,8} (4 alike) : tiiqmathlib/Float to IQN  Q_value=16
  IQN x IQN{1..6} (6 alike) : tiiqmathlib/IQN x IQN  multiplyOption=Multiply
  Sum : Sum  Inputs=+--
  Sum2 : Sum  Inputs=+-
  Alpha : Outport  VectorParamsAs1DForOutWhenUnconnected=off
  Beta : Outport  Port=2  VectorParamsAs1DForOutWhenUnconnected=off
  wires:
  Constant5/1 -> Float to IQN4/1
  Float to IQN3/1 -> IQN x IQN2/1, IQN x IQN1/1
  IQN x IQN3/1 -> Sum2/1
  Sum/1 -> IQN x IQN5/2
  IQN x IQN5/1 -> Alpha/1
  IQN x IQN1/1 -> Sum/2
  Constant8/1 -> Float to IQN5/1
  Constant9/1 -> Float to IQN8/1
  Float to IQN5/1 -> IQN x IQN4/2
  IQN x IQN4/1 -> Sum2/2
  Float to IQN8/1 -> IQN x IQN6/2, IQN x IQN5/1
  IQN x IQN2/1 -> Sum/3
  Float to IQN4/1 -> IQN x IQN3/1
  Constant4/1 -> Float to IQN3/1
  ABC/1 -> Demux/1
  Demux/2 -> IQN x IQN1/2, IQN x IQN3/2
  Demux/3 -> IQN x IQN2/2, IQN x IQN4/1
  Demux/1 -> Sum/1
  Sum2/1 -> IQN x IQN6/1
  IQN x IQN6/1 -> Beta/1

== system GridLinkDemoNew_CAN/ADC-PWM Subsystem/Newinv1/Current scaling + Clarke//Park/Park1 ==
  Alpha : Inport
  Beta : Inport  Port=2
  theta : Inport  Port=3
  Product{,1..3} (4 alike) : Product
  Sum2 : Sum  Inputs=|++
  Sum3 : Sum  Inputs=|+-
  cos IQN1 : tiiqmathlib/Trig Fcn IQN  functionOption=_IQcosPU
  sin IQN1 : tiiqmathlib/Trig Fcn IQN  functionOption=_IQsinPU
  d : Outport  VectorParamsAs1DForOutWhenUnconnected=off
  q : Outport  Port=2  VectorParamsAs1DForOutWhenUnconnected=off
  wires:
  Product3/1 -> Sum3/2
  sin IQN1/1 -> Product3/2, Product1/2
  Product2/1 -> Sum3/1
  cos IQN1/1 -> Product2/2, Product/2
  theta/1 -> sin IQN1/1, cos IQN1/1
  Sum2/1 -> d/1
  Product/1 -> Sum2/1
  Alpha/1 -> Product3/1, Product/1
  Product1/1 -> Sum2/2
  Beta/1 -> Product2/1, Product1/1
  Sum3/1 -> q/1

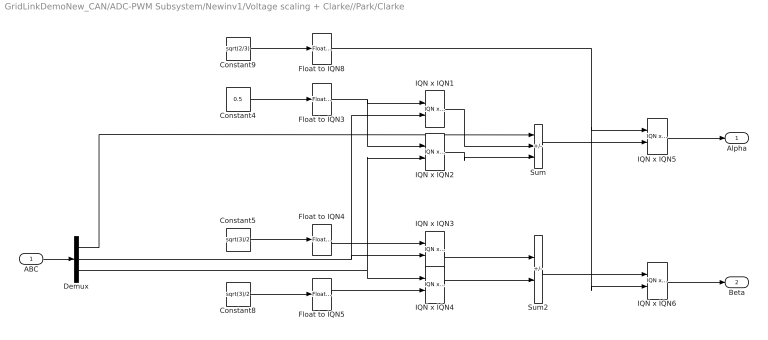
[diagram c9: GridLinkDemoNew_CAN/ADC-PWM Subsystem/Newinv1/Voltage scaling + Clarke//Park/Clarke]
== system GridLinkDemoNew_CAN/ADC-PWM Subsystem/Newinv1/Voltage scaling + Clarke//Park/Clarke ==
  ABC : Inport
  Constant4 : Constant  Value=0.5  OutDataTypeStr=single
  Constant5 : Constant  Value=sqrt(3)/2  OutDataTypeStr=single
  Constant8 : Constant  Value=sqrt(3)/2  OutDataTypeStr=single
  Constant9 : Constant  Value=sqrt(2/3)  OutDataTypeStr=single
  Demux : Demux  Outputs=3
  Float to IQN{3..5,8} (4 alike) : tiiqmathlib/Float to IQN  Q_value=16
  IQN x IQN{1..6} (6 alike) : tiiqmathlib/IQN x IQN  multiplyOption=Multiply
  Sum : Sum  Inputs=+--
  Sum2 : Sum  Inputs=+-
  Alpha : Outport  VectorParamsAs1DForOutWhenUnconnected=off
  Beta : Outport  Port=2  VectorParamsAs1DForOutWhenUnconnected=off
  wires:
  Constant5/1 -> Float to IQN4/1
  Float to IQN3/1 -> IQN x IQN2/1, IQN x IQN1/1
  IQN x IQN3/1 -> Sum2/1
  Sum/1 -> IQN x IQN5/2
  IQN x IQN5/1 -> Alpha/1
  IQN x IQN1/1 -> Sum/2
  Constant8/1 -> Float to IQN5/1
  Constant9/1 -> Float to IQN8/1
  Float to IQN5/1 -> IQN x IQN4/2
  IQN x IQN4/1 -> Sum2/2
  Float to IQN8/1 -> IQN x IQN6/2, IQN x IQN5/1
  IQN x IQN2/1 -> Sum/3
  Float to IQN4/1 -> IQN x IQN3/1
  Constant4/1 -> Float to IQN3/1
  ABC/1 -> Demux/1
  Demux/2 -> IQN x IQN1/2, IQN x IQN3/2
  Demux/3 -> IQN x IQN2/2, IQN x IQN4/1
  Demux/1 -> Sum/1
  Sum2/1 -> IQN x IQN6/1
  IQN x IQN6/1 -> Beta/1

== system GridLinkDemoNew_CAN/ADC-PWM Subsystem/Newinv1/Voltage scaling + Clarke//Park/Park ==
  Alpha : Inport
  Beta : Inport  Port=2
  theta : Inport  Port=3
  Product{,1..3} (4 alike) : Product
  Sum2 : Sum  Inputs=|++
  Sum3 : Sum  Inputs=|+-
  cos IQN1 : tiiqmathlib/Trig Fcn IQN  functionOption=_IQcosPU
  sin IQN1 : tiiqmathlib/Trig Fcn IQN  functionOption=_IQsinPU
  d : Outport  VectorParamsAs1DForOutWhenUnconnected=off
  q : Outport  Port=2  VectorParamsAs1DForOutWhenUnconnected=off
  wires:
  Product3/1 -> Sum3/2
  sin IQN1/1 -> Product3/2, Product1/2
  Product2/1 -> Sum3/1
  cos IQN1/1 -> Product2/2, Product/2
  theta/1 -> sin IQN1/1, cos IQN1/1
  Sum2/1 -> d/1
  Product/1 -> Sum2/1
  Alpha/1 -> Product3/1, Product/1
  Product1/1 -> Sum2/2
  Beta/1 -> Product2/1, Product1/1
  Sum3/1 -> q/1

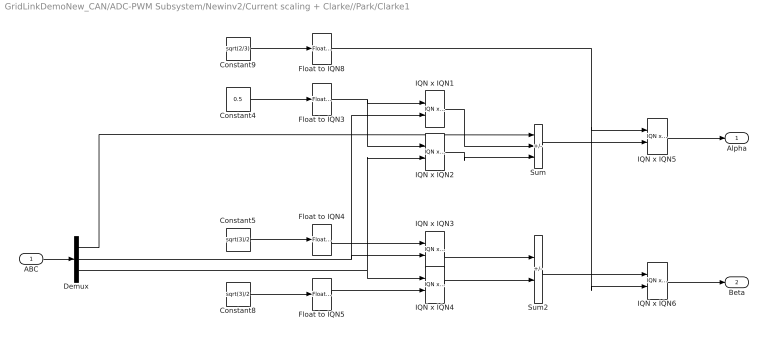
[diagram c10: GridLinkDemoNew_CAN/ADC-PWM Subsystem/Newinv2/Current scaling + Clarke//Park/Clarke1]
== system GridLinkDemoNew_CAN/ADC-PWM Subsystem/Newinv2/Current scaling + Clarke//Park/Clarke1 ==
  ABC : Inport
  Constant4 : Constant  Value=0.5  OutDataTypeStr=single
  Constant5 : Constant  Value=sqrt(3)/2  OutDataTypeStr=single
  Constant8 : Constant  Value=sqrt(3)/2  OutDataTypeStr=single
  Constant9 : Constant  Value=sqrt(2/3)  OutDataTypeStr=single
  Demux : Demux  Outputs=3
  Float to IQN{3..5,8} (4 alike) : tiiqmathlib/Float to IQN  Q_value=16
  IQN x IQN{1..6} (6 alike) : tiiqmathlib/IQN x IQN  multiplyOption=Multiply
  Sum : Sum  Inputs=+--
  Sum2 : Sum  Inputs=+-
  Alpha : Outport  VectorParamsAs1DForOutWhenUnconnected=off
  Beta : Outport  Port=2  VectorParamsAs1DForOutWhenUnconnected=off
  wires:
  Constant5/1 -> Float to IQN4/1
  Float to IQN3/1 -> IQN x IQN2/1, IQN x IQN1/1
  IQN x IQN3/1 -> Sum2/1
  Sum/1 -> IQN x IQN5/2
  IQN x IQN5/1 -> Alpha/1
  IQN x IQN1/1 -> Sum/2
  Constant8/1 -> Float to IQN5/1
  Constant9/1 -> Float to IQN8/1
  Float to IQN5/1 -> IQN x IQN4/2
  IQN x IQN4/1 -> Sum2/2
  Float to IQN8/1 -> IQN x IQN6/2, IQN x IQN5/1
  IQN x IQN2/1 -> Sum/3
  Float to IQN4/1 -> IQN x IQN3/1
  Constant4/1 -> Float to IQN3/1
  ABC/1 -> Demux/1
  Demux/2 -> IQN x IQN1/2, IQN x IQN3/2
  Demux/3 -> IQN x IQN2/2, IQN x IQN4/1
  Demux/1 -> Sum/1
  Sum2/1 -> IQN x IQN6/1
  IQN x IQN6/1 -> Beta/1

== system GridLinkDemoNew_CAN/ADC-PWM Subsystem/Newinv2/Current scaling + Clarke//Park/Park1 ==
  Alpha : Inport
  Beta : Inport  Port=2
  theta : Inport  Port=3
  Product{,1..3} (4 alike) : Product
  Sum2 : Sum  Inputs=|++
  Sum3 : Sum  Inputs=|+-
  cos IQN1 : tiiqmathlib/Trig Fcn IQN  functionOption=_IQcosPU
  sin IQN1 : tiiqmathlib/Trig Fcn IQN  functionOption=_IQsinPU
  d : Outport  VectorParamsAs1DForOutWhenUnconnected=off
  q : Outport  Port=2  VectorParamsAs1DForOutWhenUnconnected=off
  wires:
  Product3/1 -> Sum3/2
  sin IQN1/1 -> Product3/2, Product1/2
  Product2/1 -> Sum3/1
  cos IQN1/1 -> Product2/2, Product/2
  theta/1 -> sin IQN1/1, cos IQN1/1
  Sum2/1 -> d/1
  Product/1 -> Sum2/1
  Alpha/1 -> Product3/1, Product/1
  Product1/1 -> Sum2/2
  Beta/1 -> Product2/1, Product1/1
  Sum3/1 -> q/1

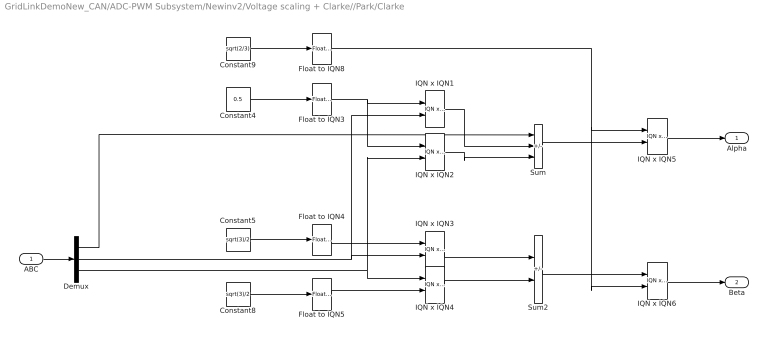
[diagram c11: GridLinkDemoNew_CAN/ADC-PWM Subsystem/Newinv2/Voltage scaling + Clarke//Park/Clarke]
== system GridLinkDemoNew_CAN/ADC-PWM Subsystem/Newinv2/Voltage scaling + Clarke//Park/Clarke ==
  ABC : Inport
  Constant4 : Constant  Value=0.5  OutDataTypeStr=single
  Constant5 : Constant  Value=sqrt(3)/2  OutDataTypeStr=single
  Constant8 : Constant  Value=sqrt(3)/2  OutDataTypeStr=single
  Constant9 : Constant  Value=sqrt(2/3)  OutDataTypeStr=single
  Demux : Demux  Outputs=3
  Float to IQN{3..5,8} (4 alike) : tiiqmathlib/Float to IQN  Q_value=16
  IQN x IQN{1..6} (6 alike) : tiiqmathlib/IQN x IQN  multiplyOption=Multiply
  Sum : Sum  Inputs=+--
  Sum2 : Sum  Inputs=+-
  Alpha : Outport  VectorParamsAs1DForOutWhenUnconnected=off
  Beta : Outport  Port=2  VectorParamsAs1DForOutWhenUnconnected=off
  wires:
  Constant5/1 -> Float to IQN4/1
  Float to IQN3/1 -> IQN x IQN2/1, IQN x IQN1/1
  IQN x IQN3/1 -> Sum2/1
  Sum/1 -> IQN x IQN5/2
  IQN x IQN5/1 -> Alpha/1
  IQN x IQN1/1 -> Sum/2
  Constant8/1 -> Float to IQN5/1
  Constant9/1 -> Float to IQN8/1
  Float to IQN5/1 -> IQN x IQN4/2
  IQN x IQN4/1 -> Sum2/2
  Float to IQN8/1 -> IQN x IQN6/2, IQN x IQN5/1
  IQN x IQN2/1 -> Sum/3
  Float to IQN4/1 -> IQN x IQN3/1
  Constant4/1 -> Float to IQN3/1
  ABC/1 -> Demux/1
  Demux/2 -> IQN x IQN1/2, IQN x IQN3/2
  Demux/3 -> IQN x IQN2/2, IQN x IQN4/1
  Demux/1 -> Sum/1
  Sum2/1 -> IQN x IQN6/1
  IQN x IQN6/1 -> Beta/1

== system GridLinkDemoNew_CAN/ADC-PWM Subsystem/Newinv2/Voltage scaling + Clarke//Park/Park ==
  Alpha : Inport
  Beta : Inport  Port=2
  theta : Inport  Port=3
  Product{,1..3} (4 alike) : Product
  Sum2 : Sum  Inputs=|++
  Sum3 : Sum  Inputs=|+-
  cos IQN1 : tiiqmathlib/Trig Fcn IQN  functionOption=_IQcosPU
  sin IQN1 : tiiqmathlib/Trig Fcn IQN  functionOption=_IQsinPU
  d : Outport  VectorParamsAs1DForOutWhenUnconnected=off
  q : Outport  Port=2  VectorParamsAs1DForOutWhenUnconnected=off
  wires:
  Product3/1 -> Sum3/2
  sin IQN1/1 -> Product3/2, Product1/2
  Product2/1 -> Sum3/1
  cos IQN1/1 -> Product2/2, Product/2
  theta/1 -> sin IQN1/1, cos IQN1/1
  Sum2/1 -> d/1
  Product/1 -> Sum2/1
  Alpha/1 -> Product3/1, Product/1
  Product1/1 -> Sum2/2
  Beta/1 -> Product2/1, Product1/1
  Sum3/1 -> q/1
